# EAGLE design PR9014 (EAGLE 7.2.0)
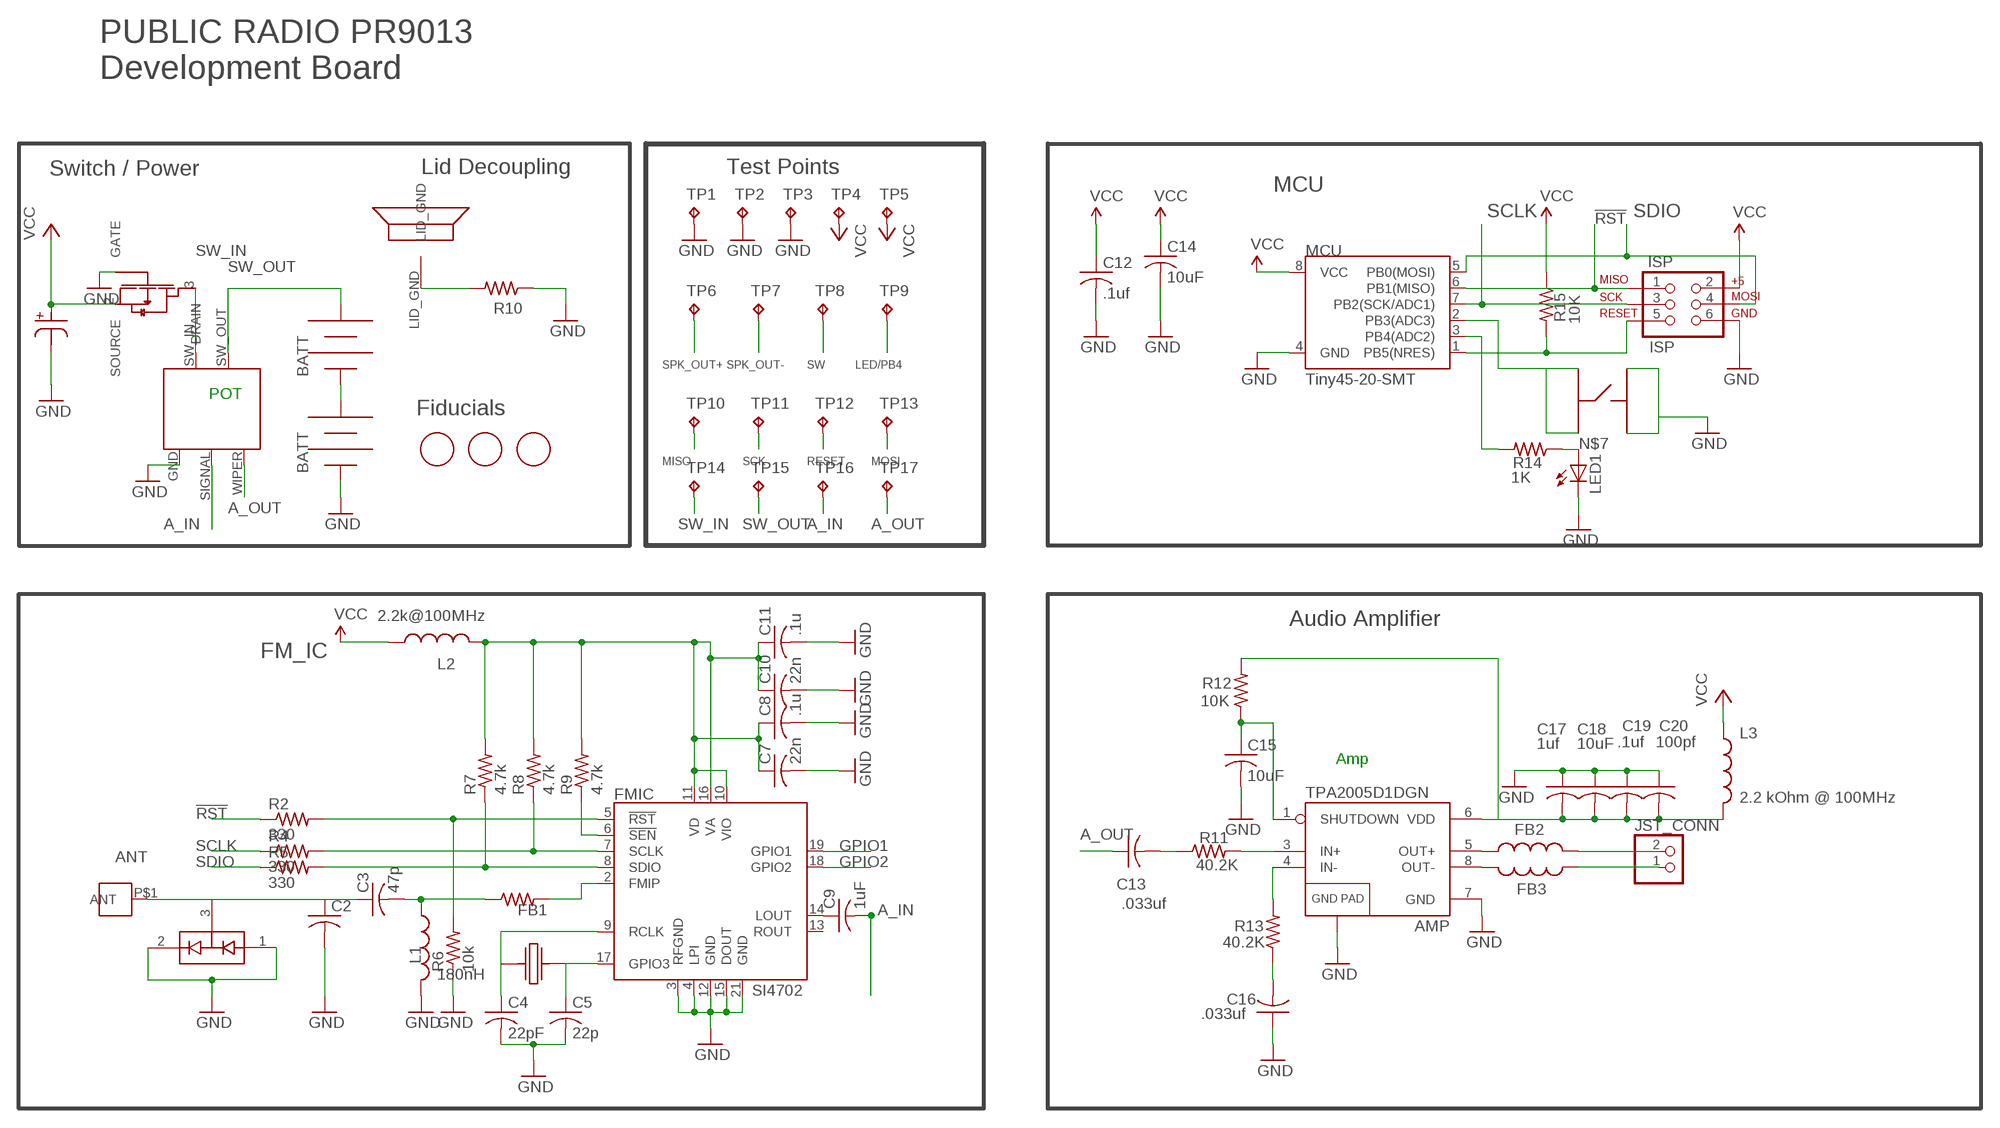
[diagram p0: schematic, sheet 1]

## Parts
AMP  TPA2005D1DGN  [POWER-SOP8]
C1  220uF  NICHICON_SERIESUD  [NICHICON_SERIESUD]
C2  C-USC0402  [C0402]
C3  47p  C-USC0402  [C0402]
C4  22pF  C-USC0402  [C0402]
C5  22p  C-USC0402  [C0402]
C7  22n  C-USC0402  [C0402]
C8  .1u  C-USC0402  [C0402]
C9  1uF  C-USC0402  [C0402]
C10  22n  C-USC0402  [C0402]
C11  .1u  C-USC0402  [C0402]
C12  .1uf  C-USC0402  [C0402]
C13  .033uf  C-USC0402  [C0402]
C14  10uF  C-USC0603  [C0603]
C15  10uF  C-USC0603  [C0603]
C16  .033uf  C-USC0402  [C0402]
C17  1uf  C-USC0402  [C0402]
C18  10uF  C-USC0603  [C0603]
C19  .1uf  C-USC0402  [C0402]
C20  100pf  C-USC0402  [C0402]
D1  BAV99  [SOT23]
FB1  R-US_R0402  [R0402]
FB2  INDUCTOR0805  [0805]
FB3  INDUCTOR0805  [0805]
FET2  AO3435  [AO3435]
FMIC  SI4702  SI470X  [SI470X]
ISP  ISP  AVR_SPI_PRG_6NS  [2X3-NS]
J1  M3_SCREW_POST  [M3_SCREW_POST]
JP5  BK-92_MPD_AA_BATT_CLIP  [BK-92_MPD_AA_BATT_CLIP]
JP6  BK-92_MPD_AA_BATT_CLIP  [BK-92_MPD_AA_BATT_CLIP]
JST_CONN  JST_2PIN-SMT-RA  [JST-PH-2-SMT-RA]
L1  180nH  INDUCTOR0805  [0805]
L2  2.2k@100MHz  INDUCTOR0402  [C0402]
L3  2.2 kOhm @ 100MHz  INDUCTOR0402  [C0402]
LED1  LEDSML0603  [SML0603]
MCU  Tiny45-20-SMT  ATTINY45TINY85-20-SMT  [SO08-EIAJ]
R1  RV170SF_TAIWANA_POT_SW  [RV170SF_TAIWANA_POT_SW]
R2  330  R-US_R0402  [R0402]
R4  330  R-US_R0402  [R0402]
R5  330  R-US_R0402  [R0402]
R6  10k  R-US_R0402  [R0402]
R7  4.7k  R-US_R0402  [R0402]
R8  4.7k  R-US_R0402  [R0402]
R9  4.7k  R-US_R0402  [R0402]
R10  R-US_R0805  [R0805]
R11  40.2K  R-US_R0402  [R0402]
R12  10K  R-US_R0402  [R0402]
R13  40.2K  R-US_R0402  [R0402]
R14  1K  R-US_R0402  [R0402]
R15  10K  R-US_R0402  [R0402]
SW1  C&K_PTS645  [C&K_TACTILE_SWITCH]
TP1  TPTP20R  [TP20R]
TP2  TPTP20R  [TP20R]
TP3  TPTP20R  [TP20R]
TP4  TPTP20R  [TP20R]
TP5  TPTP20R  [TP20R]
TP6  TPTP20R  [TP20R]
TP7  TPTP20R  [TP20R]
TP8  TPTP20R  [TP20R]
TP9  TPTP20R  [TP20R]
TP10  TPTP20R  [TP20R]
TP11  TPTP20R  [TP20R]
TP12  TPTP20R  [TP20R]
TP13  TPTP20R  [TP20R]
TP14  TPTP20R  [TP20R]
TP15  TPTP20R  [TP20R]
TP16  TPTP20R  [TP20R]
TP17  TPTP20R  [TP20R]
U$1  CE32A_FOR_JST  [CE32A_FOR_JST]
U$3  FIDUCIAL  [FIDUCIAL_1MM]
U$4  FIDUCIAL  [FIDUCIAL_1MM]
U$5  FIDUCIAL  [FIDUCIAL_1MM]
U$6  ABS25XTAL  [ABS25XTAL]

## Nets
3.3V: C7.1 C8.1 C10.1 C11.1 FMIC.10(VIO) FMIC.11(VD) FMIC.16(VA) L2.2 R7.2 R8.2 R9.2
!RST: ISP.1 MCU.6(PB1(MISO)) R2.1 TP10.TP
!RST-L: FMIC.5(!RST) R2.2 R6.2
!SEN-L: FMIC.6(!SEN) R9.1
A_IN: C9.2 R1.SIGNAL TP16.TP
A_OUT: C13.1 R1.WIPER TP17.TP
ANT [antenna]: C2.1 C3.1 D1.3(COM) J1.P$1(ANT)
GND: AMP.7(GND) AMP.9(GND) C1.P$2 C2.2 C4.2 C5.2 C7.2 C8.2 C10.2 C11.2 C12.2 C14.2 C15.2 C16.1 C17.1 C18.1 C19.1 C20.1 D1.1(A1) D1.2(C2) FET2.1(GATE) FMIC.3(RFGND) FMIC.4(LPI) FMIC.12(GND) FMIC.15(DOUT) FMIC.21(GND) ISP.6 JP6.NEG JP6.NEG@2(NEG) L1.2 LED1.C MCU.4(GND) R1.GND R6.1 R10.1 SW1.P$1 SW1.P$2 TP1.TP TP2.TP TP3.TP
GPIO1: FMIC.19(GPIO1)
GPIO2: FMIC.18(GPIO2)
LED/PB4: MCU.3(PB4(ADC2)) R14.2 TP9.TP
N$1: C4.1 FMIC.9(RCLK) U$6.P$1
N$3: C13.2 R11.1
N$4: AMP.3(IN+) R11.2
N$5: AMP.4(IN-) R13.2
N$6: FB1.2 FMIC.2(FMIP)
N$7: LED1.A R14.1
N$8: R10.2 U$1.LID_GND
N$9: C9.1 FMIC.14(LOUT)
N$10: C5.1 FMIC.17(GPIO3) U$6.P$4
N$13: JP5.NEG JP5.NEG@2(NEG) JP6.POS JP6.POS@2(POS)
N$16 [antenna]: C3.2 FB1.1 L1.1
N$17: AMP.8(OUT-) FB3.2
N$18: AMP.6(VDD) C17.2 C18.2 C19.2 C20.2 L3.2 R12.2
N$19: AMP.5(OUT+) FB2.1
N$20: AMP.1(SHUTDOWN) C15.1 R12.1
N$23: C16.2 R13.1
RESET: ISP.5 MCU.1(PB5(NRES)) R15.2 TP12.TP
SCLK: ISP.3 MCU.7(PB2(SCK/ADC1)) R4.1 TP11.TP
SCLK-L: FMIC.7(SCLK) R4.2 R8.1
SDIO: ISP.4 MCU.5(PB0(MOSI)) R5.1 TP13.TP
SDIO-L: FMIC.8(SDIO) R5.2 R7.1
SPK_OUT+: FB2.2 JST_CONN.2 TP6.TP
SPK_OUT-: FB3.1 JST_CONN.1 TP7.TP
SW: MCU.2(PB3(ADC3)) SW1.P$3 SW1.P$4 TP8.TP
SW_IN: FET2.3(DRAIN) R1.SW_IN TP14.TP
SW_OUT: JP5.POS JP5.POS@2(POS) R1.SW_OUT TP15.TP
VCC: C1.P$1 C12.1 C14.1 FET2.2(SOURCE) ISP.2 L2.1 L3.1 MCU.8(VCC) R15.1 TP4.TP TP5.TP
Unconnected: FMIC.13(ROUT)

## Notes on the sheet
- PUBLIC RADIO PR9013
  Development Board
- Switch / Power | Lid Decoupling | Test Points
- MCU
- POT
- Fiducials
- MISO | SCK | RESET | MOSI
- Audio Amplifier
- FM_IC
- Amp

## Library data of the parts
AMP = PR_Parts_Library:TPA2005D1: 1.4W MONO CLASS-D AUDIO POWER AMPLIFIER The TPA2005D1 is a 1.4-W high efficiency filter-free class-D audio power amplifier in a BGA, QFN, or MSOP package that requires only three external components. Datasheet: http://focus.ti.com/lit/ds/symlink/tpa2005d1.pdf 1.4 W Into 8 ? From a 5V Supply at THD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
C1 = PR_Parts_Library:NICHICON_SERIESUD: Nichicon UD Series 220uf Cap
C2-C5 C7-C20 = resistor:C-US: CAPACITOR, American symbol
D1 = SparkFun-DiscreteSemi:BAV99: Two small signal silicon diodes connected anode to cathode. Connections to all three nodes available. DIO-10647; PROD_ID: DIO-10647
FB1 R2 R4-R15 = resistor:R-US_: RESISTOR, American symbol
FB2 FB3 L1-L3 = SparkFun-Passives:INDUCTOR: Inductors
FET2 = PR_Parts_Library:AO3435: MOSFET P-CH 20V 2.9A SOT23 MFG # AO3435
FMIC = PR_Parts_Library:SI470X: SI4702-C19-GMR
ISP = SparkFun-Connectors:AVR_SPI_PRG_6: AVR ISP 6 Pin This is the reduced ISP connector for AVR programming. Common on Arduino. This footprint will take up less PCB space and can be used with a 10-pin to 6-pin adapter such as SKU: BOB-08508
J1 = PR_Parts_Library:M3_SCREW_POST
JP5 JP6 = PR_Parts_Library:BK-92_MPD_AA_BATT_CLIP
JST_CONN = adafruit:JST_2PIN: JST 2-Pin Connectors of various flavors
LED1 = led:LED: LED
MCU = SparkFun-DigitalIC:ATTINY45: Atmel 8-pin 2/4/8kB flash uC; PROD_ID: IC-09092; VALUE: Tiny85-20-SMT
R1 = PR_Parts_Library:RV170SF_TAIWANA_POT_SW
SW1 = PR_Parts_Library:C&K_PTS645: 6MM Tactile Switch MFG# PTS645SM43SMTR92 LFS
TP1-TP17 = testpad:TP: Test pad
U$1 = PR_Parts_Library:CE32A_FOR_JST: This package allows one of the speaker screws to be used as a ground terminal for The Public Radio's lid.
U$3-U$5 = adafruit:FIDUCIAL: For use by pick and place machines to calibrate the vision/machine, 1mm
U$6 = PR_Parts_Library:ABS25XTAL: 4PIN 32.768 Xtal

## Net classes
1 antenna: clearance 1.27 mm

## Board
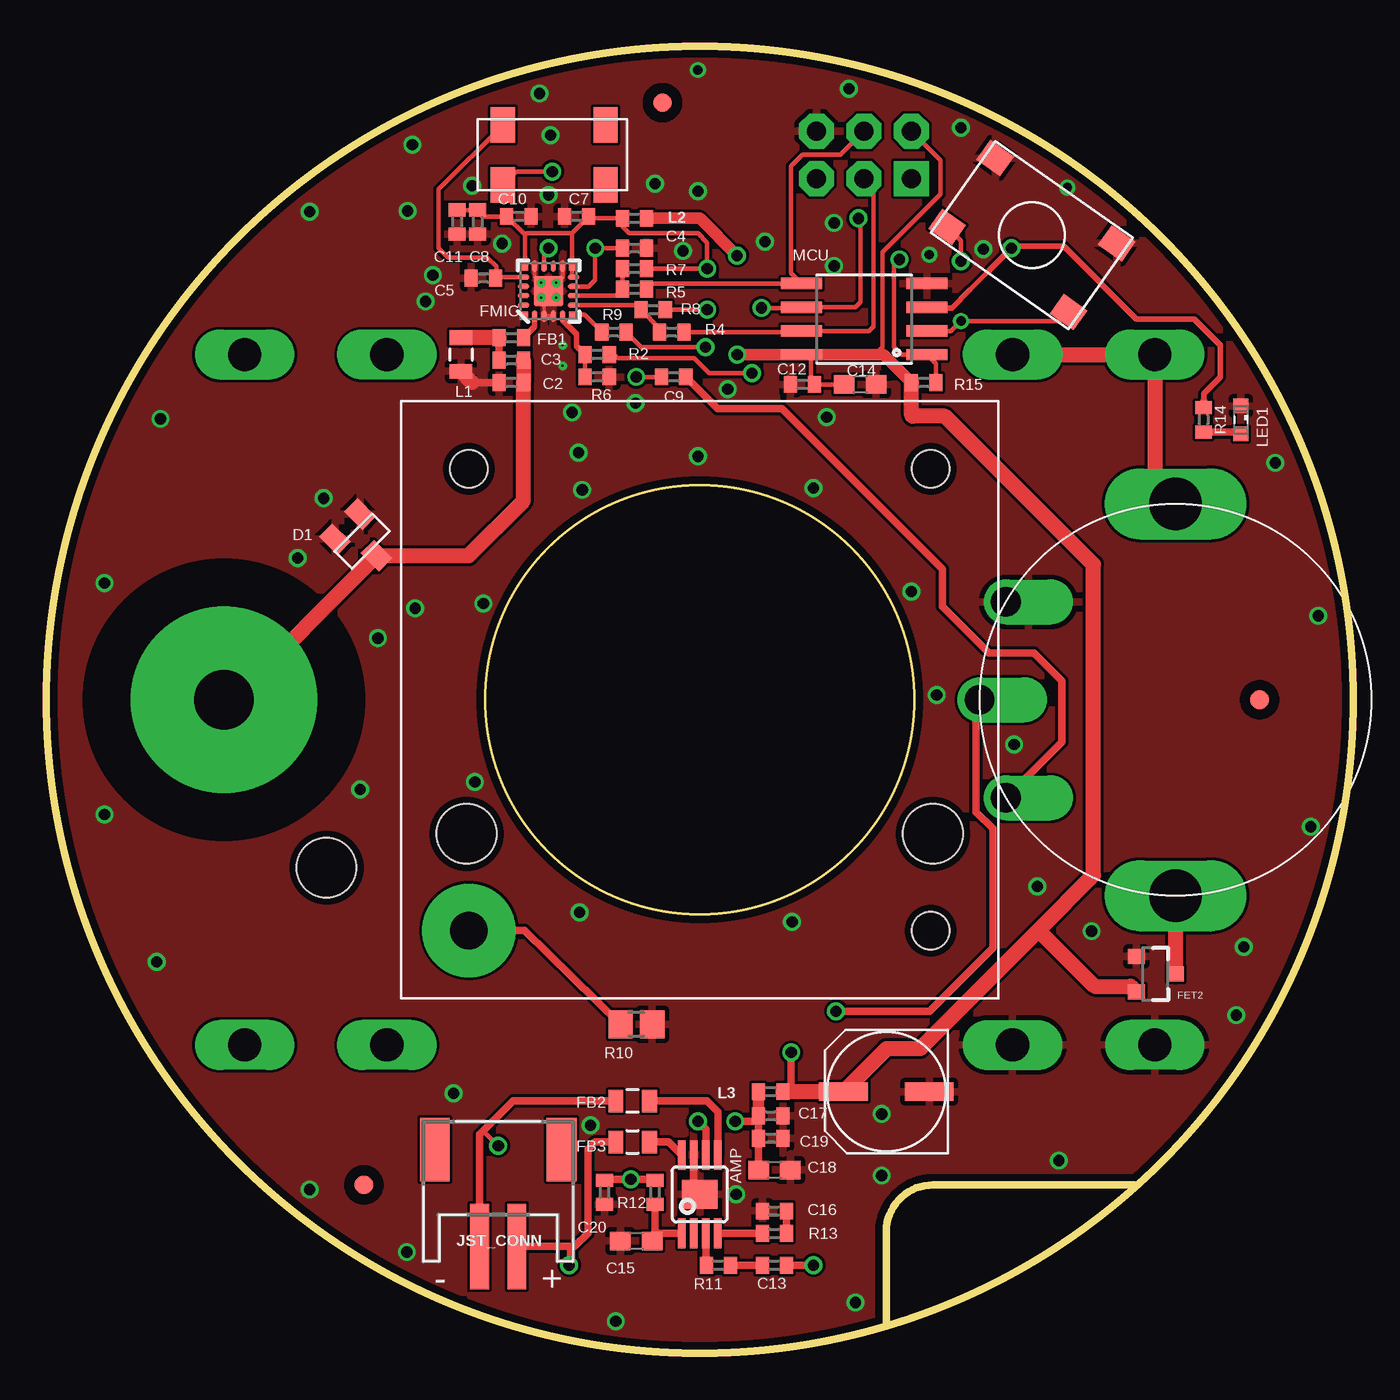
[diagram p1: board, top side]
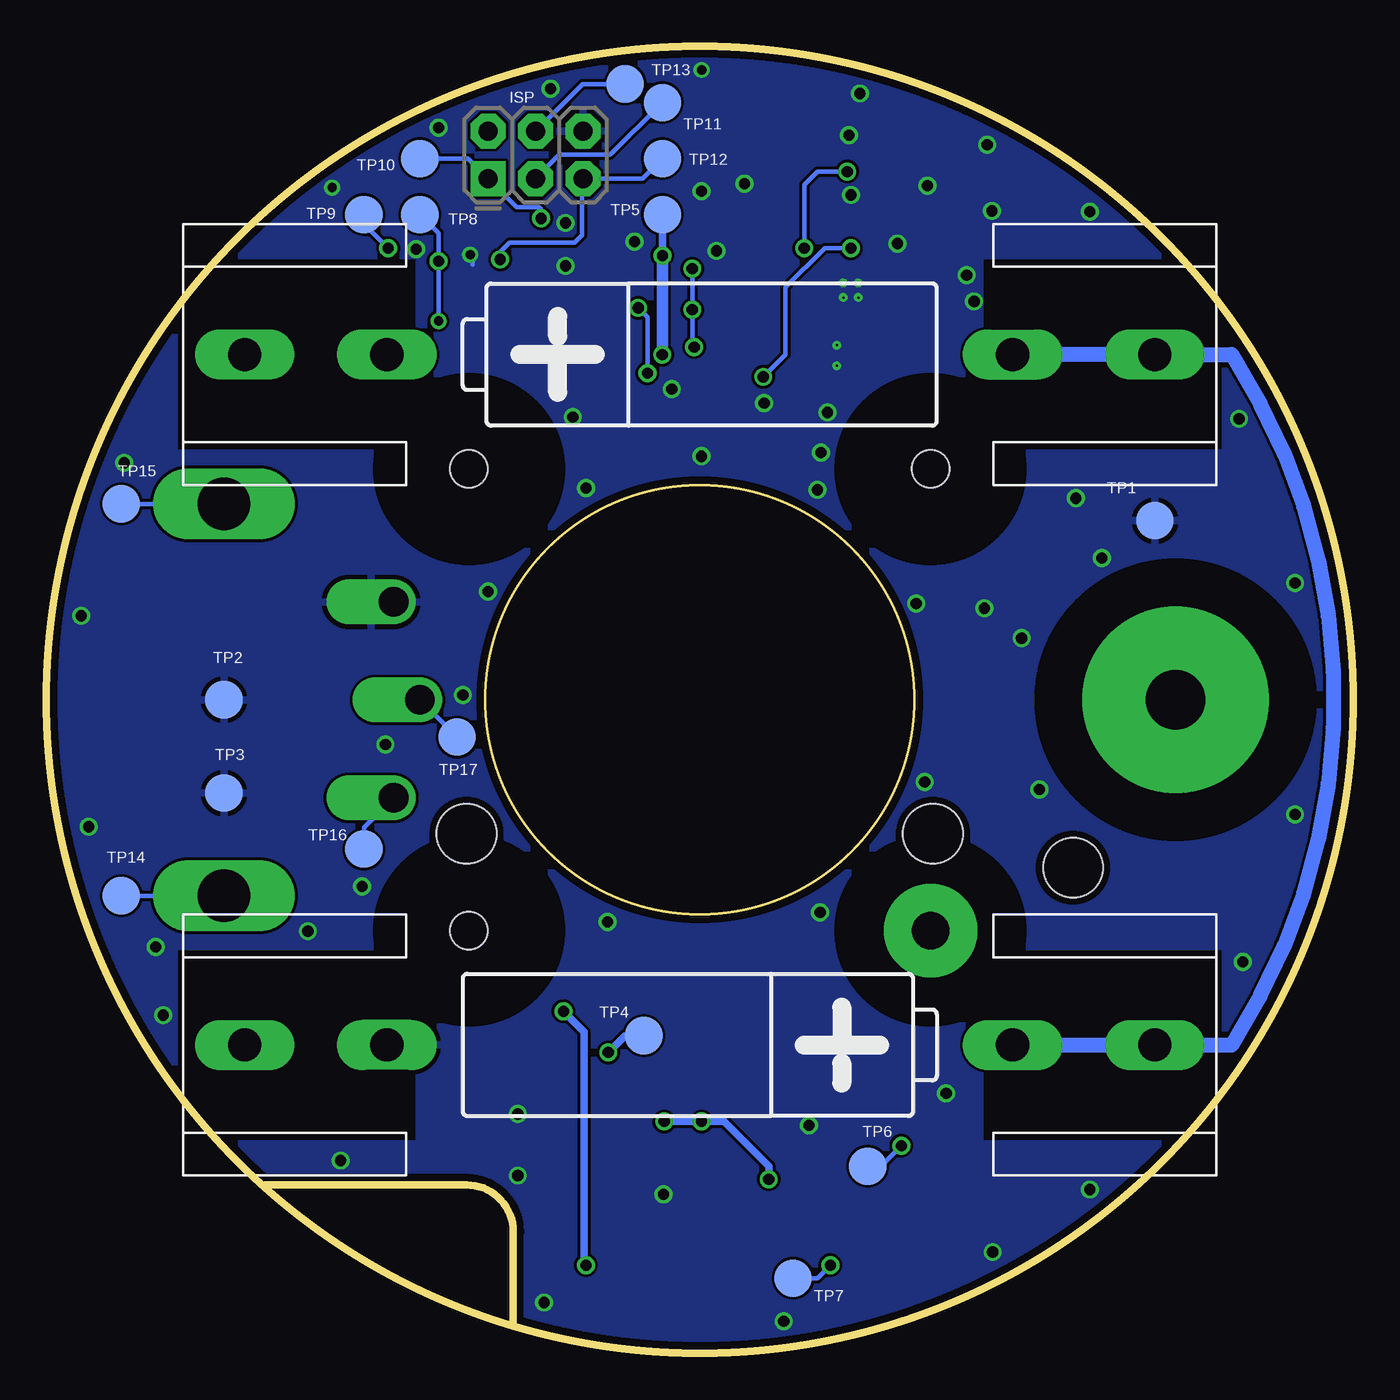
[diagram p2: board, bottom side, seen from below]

Size 70 x 70 mm. Coordinates in mm from the lower left corner, seen from the top.
Outline: 45,1.5 45,6.5 arc-90 47.5,9 58.3,9
Outline: circle at 35,35 radius 35
Copper layers (1*16): Top 0.0356mm / dielectric 1.5011mm / Bottom 0.0356mm
Design rules "LaenPCBOrder": minimum track width 6mil, minimum drill 13mil, track to track 6mil, track to pad 6mil, pad to pad 6mil, via to via 6mil, smd to smd 6mil, copper to edge 15mil, drill to drill 6mil, minimum pad ring 7mil, minimum via ring 7mil, stop-mask expansion 3mil, vias tented up to drill 0mil, thermal gap 10mil
Holes 3.2 mm at 15,26

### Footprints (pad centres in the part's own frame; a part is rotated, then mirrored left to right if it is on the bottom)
POWER-SOP8 = smd 0.4 x 1.6: 1 -0.975,-2.1; 2 -0.325,-2.1; 3 0.325,-2.1; 4 0.975,-2.1; 5 0.975,2.1; 6 0.325,2.1; 7 -0.325,2.1; 8 -0.975,2.1 | smd 1.89 x 1.57: 9 0,0
NICHICON_SERIESUD = smd 1 x 2.6: P$1 0,2.3; P$2 0,-2.3
C0402 = smd 0.7 x 0.9: 1 -0.65,0; 2 0.65,0
C0603 = smd 1.1 x 1: 1 -0.85,0; 2 0.85,0
SOT23 = smd 1 x 1.4: 1 -0.95,-1.1; 2 0.95,-1.1; 3 0,1.1
R0402 = smd 0.7 x 0.9: 1 -0.65,0; 2 0.65,0
0805 = smd 0.8 x 1.2: 1 -0.9,0; 2 0.9,0
AO3435 = smd 0.8 x 0.9: 1 -0.95,-1; 2 0.95,-1; 3 0,1.1
SI470X = smd 0.34 x 0.34: 1 -1.275,1.265; 6 -1.265,-1.265; 11 1.265,-1.265; 16 1.265,1.265 | smd 0.61 x 0.28: 2 -1.335,0.75; 3 -1.335,0.25; 4 -1.335,-0.25; 5 -1.335,-0.75; 12 1.335,-0.75; 13 1.335,-0.25; 14 1.335,0.25; 15 1.335,0.75 | smd 0.28 x 0.61: 7 -0.75,-1.335; 8 -0.25,-1.335; 9 0.25,-1.335; 10 0.75,-1.335; 17 0.75,1.335; 18 0.25,1.335; 19 -0.25,1.335; 20 -0.75,1.335 | smd 1.6 x 1.6: 21 0,0
2X3-NS = drill 1.016 pad 1.88 square: 1 -2.54,-1.27 | drill 1.016 pad 1.88 octagon: 2 -2.54,1.27; 3 0,-1.27; 4 0,1.27; 5 2.54,-1.27; 6 2.54,1.27
M3_SCREW_POST = drill 3.2 pad 10: P$1 0,0
BK-92_MPD_AA_BATT_CLIP = drill 1.778 long: NEG -24.384,0; NEG@2 -16.764,0; POS 16.764,0; POS@2 24.384,0
JST-PH-2-SMT-RA = smd 1 x 4.6: 1 1,-3.7; 2 -1,-3.7 | smd 1.6 x 3.4: NC1 -3.4,1.5; NC2 3.4,1.5
SML0603 = smd 0.8 x 0.8: A 0.75,0; C -0.75,0
SO08-EIAJ = smd 0.61 x 2.21: 1 -1.905,-3.378; 2 -0.635,-3.378; 3 0.635,-3.378; 4 1.905,-3.378; 5 1.905,3.353; 6 0.635,3.353; 7 -0.635,3.353; 8 -1.905,3.353
RV170SF_TAIWANA_POT_SW = drill 1.6 offset: GND -5.25,-9.09; SIGNAL 5.25,-9.09; WIPER 0,-10.5 | drill 2.8 long: SW_IN 10.5,0; SW_OUT -10.5,0
R0805 = smd 1.3 x 1.5: 1 -0.85,0; 2 0.85,0
C&K_TACTILE_SWITCH = smd 1.55 x 1.3: P$1 -3.975,2.25; P$2 3.975,2.25; P$3 -3.975,-2.25; P$4 3.975,-2.25
TP20R = smd 2 x 2: TP 0,0
CE32A_FOR_JST = drill 2 pad 5: LID_GND -12.37,-12.37 | hole 2: -12.37,12.37; 12.37,12.37; 12.37,-12.37 | hole 3.2: -12.497,-7.188; 12.497,-7.188
FIDUCIAL_1MM = smd 1 x 1: 1 0,0
ABS25XTAL = smd 1.3 x 1.9: P$1 -2.75,-1.6; P$2 2.75,-1.6; P$3 2.75,1.6; P$4 -2.75,1.6

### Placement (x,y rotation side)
AMP  35,8.5 0 top
C1  45,14 90 top
C2  24.9,52 180 top
C3  24.9,53.2 180 top
C4  31.5,59.2 0 top
C5  23.4,57.6 180 top
C7  28.4,60.9 180 top
C8  23.1,60.6 270 top
C9  33.6,52.3 0 top
C10  25.3,60.9 0 top
C11  22,60.6 270 top
C12  40.5,51.9 180 top
C13  39,4.7 180 top
C14  43.6,51.9 0 top
C15  31.6,6 180 top
C16  39,7.6 0 top
C17  38.8,12.7 180 top
C18  39,9.8 180 top
C19  38.8,11.5 180 top
C20  29.9,8.6 90 top
D1  16.9,43.5 225 top
FB1  24.9,54.4 0 top
FB2  31.4,13.5 180 top
FB3  31.4,11.3 0 top
FET2  59.4,20.3 270 top
FMIC  26.9,56.9 90 top
ISP  43.8,64.2 0 bottom
J1  9.5,35 0 top
JP5  35,53.5 180 bottom
JP6  35,16.5 0 bottom
JST_CONN  24.2,9.4 0 top
L1  22.2,53.5 270 top
L2  31.5,60.8 180 top
L3  38.8,14 180 top
LED1  64,50 270 top
MCU  43.8,55.4 90 top
R1  60.5,35 270 top
R2  29.5,53.5 180 top
R4  33.5,54.7 180 top
R5  31.5,57 180 top
R6  29.5,52.3 180 top
R7  31.5,58.1 0 top
R8  32.5,55.9 0 top
R9  30.4,54.7 0 top
R10  31.6,17.6 180 top
R11  36,4.7 180 top
R12  32.6,8.6 90 top
R13  39,6.4 180 top
R14  62,50 90 top
R15  47,52 0 top
SW1  52.8,59.9 325 top
TP1  10.6,44.6 0 bottom
TP2  60.5,35 0 bottom
TP3  60.5,30 0 bottom
TP4  38,17 0 bottom
TP5  37,61 0 bottom
TP6  26,10 0 bottom
TP7  30,4 0 bottom
TP8  50,61 0 bottom
TP9  53,61 0 bottom
TP10  50,64 0 bottom
TP11  37,67 0 bottom
TP12  37,64 0 bottom
TP13  39,68 0 bottom
TP14  66,24.5 0 bottom
TP15  66,45.5 0 bottom
TP16  53,27 0 bottom
TP17  48,33 0 bottom
U$1  35,35 0 top
U$3  17,9 0 top
U$4  33,67 0 top
U$5  65,35 0 top
U$6  27.2,64.2 0 top

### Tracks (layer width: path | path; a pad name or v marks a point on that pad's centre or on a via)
3.3V  (via drill 0.6)
  Top 0.254: FMIC.10 28.16,57.72 FMIC.11 28.16,60.02 | 34.35,58.1 R7.2 v35.4,58.1 35.4,59.5 34.9,60 31.2,60 30.85,60.35 L2.2 29.15,60.8 C7.1 28.16,60.02 | R9.2 31.85,53.9 v35.3,53.9 | FMIC.16 25.64,59.91 | 25.64,59.91 C10.1 23.45,60.9 C8.1 C11.1 | 28.16,60.02 25.73,60.02 25.64,59.91 | R8.2 v35.4,55.9
  Bottom 0.254: v35.3,53.9 35.4,54 v35.4,55.9 v35.4,58.1
!RST  (via drill 0.6)
  Top 0.254: MCU.6 41,56.03 | 41,56.03 43.34,56.03 43.6,56.3 43.6,60.7 v43.5,60.8 | v38.3,56 40.97,56 41,56.03 | R2.1 30.4,53.5 30.6,53.3 34.7,53.3 35.5,52.5 v37.8,52.5
  Bottom 0.254: v43.5,60.8 43.5,61.3 43.6,61.4 44.81,61.4 ISP.1 47.41,64 TP10.TP | v37.8,52.5 37.8,55.5 v38.3,56
!RST-L
  Top 0.254: R6.2 R2.2
  Top 0.305: FMIC.5 27.65,55.35 28.4,54.6 28.4,53.95 R2.2
!SEN-L
  Top 0.254: FMIC.6 28.82,55.63 R9.1
A_IN
  Top 0.406: R1.SIGNAL 54.4,32.74 54.4,36 52.9,37.5 50.5,37.5 48,40 48,42 39.4,50.6 35.95,50.6 C9.2
  Bottom 0.254: TP16.TP 53,28.16 R1.SIGNAL
A_OUT  (via drill 0.6)
  Top 0.406: R1.WIPER 49.8,34.8 49.8,29 50.7,28.1 50.7,21.7 47.3,18.3 v42.3,18.3 | C13.1 v41.1,4.7
  Bottom 0.254: TP17.TP R1.WIPER
  Bottom 0.406: v42.3,18.3 41.2,17.2 41.2,4.8 v41.1,4.7
ANT
  Top 0.813: J1.P$1 9.96,35 D1.3 22.62,42.72 25.55,45.65 C2.1 C3.1
GND  (via drill 0.1, 0.5, 0.6)
  Top 0.2: FMIC.15 26.15,57.65 26.2,57.65 v26.5,57.35 | FMIC.3 26.65,56.4 v26.5,56.55 | 27.65,57.65 27.6,57.65 v27.3,57.35
  Top 0.254: FMIC.12 27.65,57.65 | C10.2 26.05,60.8 | FMIC.3 FMIC.4
  Top 0.406: AMP.7 34.67,8.82 AMP.9 | C2.2 22.8,52
  Top 0.813: 22.8,52 L1.2
  Bottom 0.254: 47.18,58.84 47.18,58.33
  other vias: 34.9,68.75 31.55,50.9 27.65,54 65.85,47.7 28.7,46.25 26.41,67.49 53.1,25 46.35,40.8 43.35,2.7 19.3,5.4 21.8,13.9 28.55,23.6 39.95,23.1 64.15,21.75 51.85,32.6 26.9,62.05 19.6,64.75 47.3,58.85 43,67.75 49,65.65 41.1,46.35 36.95,8.5 29.15,12.2 44.75,12.8 41.8,50.15 56,22.6 54.7,62.45 38.5,59.55 47.7,35.25 20.7,57.75 27.3,56.55 27,65.25 42.2,60.55 42.2,58.25 32.6,62.65 34.1,59.05 24.4,59.45 22.8,62.55 36.5,51.65 50.2,59.15 14.1,61.15 6.1,50.05 3.1,41.25 3.1,28.85 14.1,8.75 30.5,1.7 44.75,9.5 54.25,10.3 63.75,18.1 67.75,28.2 68.15,39.5 27.65,52.9 19.35,61.2 28.15,50.4 19.75,39.9 23.4,40.15 22.95,30.6 34.9,48.05 20.3,56.35 16.8,30.2 5.9,20.95 34.9,62.25 28.5,48.25 17.75,38.3 13.45,42.6 14.85,45.8
  pour Bottom: 0,35 arc90 35,0 arc90 70,35 arc90 35,70 arc90
  pour Top: 0,35 arc90 35,0 arc90 70,35 arc90 35,70 arc90
LED/PB4  (via drill 0.6)
  Top 0.254: 50.5,58 49.45,56.95 | 47.34,56.2 MCU.3
  Top 0.305: 50.5,58 v51.7,59.2 51.8,59.3 54.5,59.3 58.4,55.4 61.5,55.4 62.9,54 62.9,52.3 62,51.4 62,51 | 49.45,56.95 48.5,56 47.21,56 MCU.3
  Top 0.406: R14.2 62,51
  Bottom 0.254: TP9.TP 53,60.5 v51.7,59.2
N$1  (via drill 0.6)
  Top 0.254: C4.1 v29.4,59.2 29.4,57.5 29.05,57.15 FMIC.9 | v27.1,63.3 25.15,63.3 U$6.P$1
  Bottom 0.254: v29.4,59.2 29.4,62.6 28.7,63.3 v27.1,63.3
N$3
  Top 0.406: R11.1 C13.2
N$4
  Top 0.406: AMP.3 35.33,4.72 R11.2
N$5
  Top 0.406: AMP.4 R13.2
N$6
  Top 0.305: FMIC.2 26.15,55 FB1.2
N$7
  Top 0.406: R14.1 63.9,49.35 LED1.A
N$8
  Top 0.406: R10.2 25.62,22.63 U$1.LID_GND
N$9  (via drill 0.6)
  Top 0.254: C9.1 v31.6,52.3 | FMIC.14 26.65,58.95 v26.9,59.2
  Bottom 0.254: v26.9,59.2 28.3,59.2 30.4,57.1 30.4,53.5 v31.6,52.3
N$10
  Top 0.254: FMIC.17 24.1,57.65 | 24.1,57.65 C5.1 | 24.1,57.65 24.1,58.2 23.6,58.7 21.5,58.7 21,59.2 21,62.35 U$6.P$4
N$13
  Bottom 0.813: JP6.POS JP6.POS@2 6.5,16.5 arc-66 6.5,53.5 JP5.NEG JP5.NEG@2
N$16
  Top 0.406: FB1.1 C3.2
  Top 0.813: FB1.1 L1.1
N$17
  Top 0.406: AMP.8 33.33,11.3 FB3.2
N$18  (via drill 0.6, 0.6 pad 0.41)
  Top 0.406: AMP.6 35.33,11.97 v34.9,12.4 | v36.9,12.4 37.85,12.4 C17.2 C19.2 C18.2 | R12.2 32.55,9.3 v31.3,9.3 29.95,9.3 C20.2
  Top 0.61: C17.2 L3.2
  Bottom 0.406: v36.9,12.4 v34.9,12.4 33.7,12.4 31.3,10 v31.3,9.3
N$19
  Top 0.406: AMP.5 35.98,12.93 35.4,13.5 FB2.1
N$20
  Top 0.406: AMP.1 32.85,6.4 32.6,6.15 | R12.1 32.6,6.15 | 32.6,6.15 C15.1
N$21
  pour Bottom: 
N$23
  Top 0.406: R13.1 C16.2
RESET  (via drill 0.6)
  Top 0.254: R15.2 47.65,53.02 MCU.1 45.8,53.49 45.4,53.9 45.4,58.3 v45.7,58.6
  Bottom 0.254: v45.7,58.6 45.7,59 45.2,59.5 41.7,59.5 41.3,59.9 41.3,62.89 ISP.5 38.07,62.93 TP12.TP
SCLK
  Top 0.254: ISP.3 44.3,62.43 44.3,55 44.06,54.77 MCU.7 40.38,54.7 R4.1
  Bottom 0.254: ISP.3 42.53,64.2 39.8,64.2 TP11.TP
SCLK-L
  Top 0.254: FMIC.7 31.8,56.15 R8.1 32.85,54.9 R4.2
SDIO
  Top 0.254: MCU.5 | MCU.5 32.45,57.3 R5.1 | MCU.5 39.9,57.85 39.9,63.6 40.5,64.2 42.53,64.2 ISP.4
  Bottom 0.254: TP13.TP 41.27,68 ISP.4
SDIO-L
  Top 0.254: R7.1 R5.2 30.5,56.65 FMIC.8
SPK_OUT+  (via drill 0.6)
  Top 0.254: v24.2,11.1 23.4,11.9
  Top 0.406: FB2.2 25,13.5 23.4,11.9 23.2,11.7 JST_CONN.2
  Bottom 0.254: TP6.TP 25.3,10 v24.2,11.1
SPK_OUT-  (via drill 0.6)
  Top 0.254: v28,4.7 28,5.7
  Top 0.406: FB3.1 29.4,11.3 29,10.9 29,6.4 28.3,5.7 28,5.7 JST_CONN.1
  Bottom 0.254: TP7.TP 28.7,4 v28,4.7
SW  (via drill 0.5, 0.6)
  Top 0.254: MCU.2 48.47,54.77 v49,55.3 54.29,55.3 SW1.P$4 | v49,58.5 49,59.59 SW1.P$3
  Bottom 0.254: v49,55.3 v49,58.5 49,60 TP8.TP
SW_IN
  Top 0.813: FET2.3 R1.SW_IN
  Bottom 0.254: TP14.TP R1.SW_IN
SW_OUT
  Top 0.813: JP5.POS JP5.POS@2 59.38,46.62 R1.SW_OUT
  Bottom 0.254: TP15.TP R1.SW_OUT
VCC  (via drill 0.6)
  Top 0.254: 40.95,53.49 MCU.8 | 39.9,14.1 40,14 | 40.95,53.49 44.4,53.49 44.8,53.9 44.8,59 47.9,62.1 47.9,63.91 ISP.2 | C14.1 C12.1 40.95,52.09 40.95,53.49
  Top 0.406: v39.9,16.1 39.9,14.1
  Top 0.61: R15.1 44.85,53.49 40.95,53.49 | MCU.8 v37.01,53.49 | v37,58.8 35,60.8 L2.1
  Top 0.813: 53.15,22.65 46.8,16.3 45,16.3 C1.P$1 40,14 L3.1 | 53.15,22.65 56.1,25.6 56.1,42.25 48.15,50.2 46.4,50.2 46.35,50.25 R15.1 | 53.15,22.65 56.15,19.65 58.1,19.65 FET2.2
  Bottom 0.406: TP5.TP v37,58.8 | TP4.TP 39,17 v39.9,16.1
  Bottom 0.61: v37.01,53.49 v37,53.5 v37,58.8

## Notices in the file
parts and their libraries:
SparkFun-Passives: Licensing: CC v3.0 Share-Alike You are welcome to use this library for commercial purposes.
SparkFun-DigitalIC: Licensing: Creative Commons ShareAlike 4.0 International - https://creativecommons.org/licenses/by-sa/4.0
